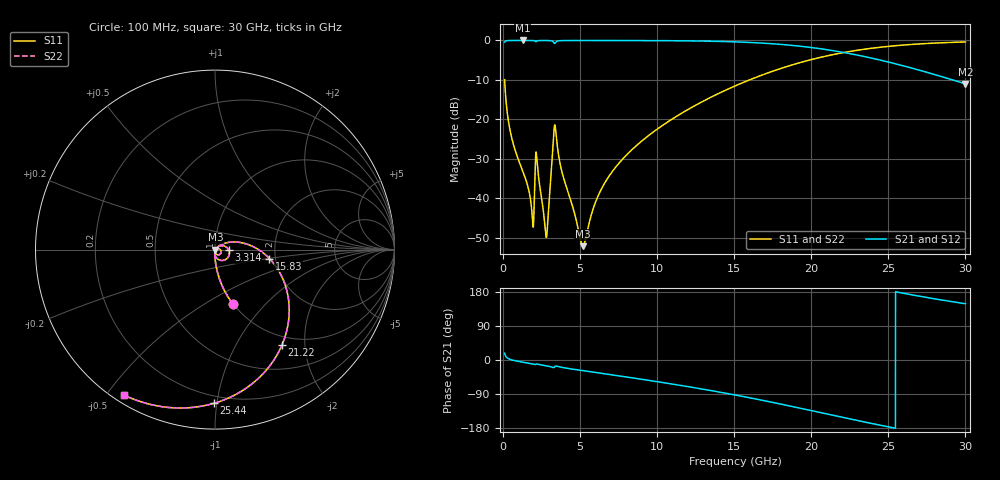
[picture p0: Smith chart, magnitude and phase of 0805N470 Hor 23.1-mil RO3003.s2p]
# GHz S MA R 50
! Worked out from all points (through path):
!   3201 points, 100 MHz to 30 GHz, reference 50 ohm
!   highest |S21| = -0.01 dB at 1.268 GHz (marker M1); lowest = -11.0 dB at 30 GHz (marker M2)
!   group delay of S21, straight-line fit = 20.5 ps
!   lowest |S11| = -52.1 dB at 5.183 GHz (marker M3), VSWR 1.00, Z = 50.2 - j0.114 ohm
!   |S11| at or under -10 dB: 100.6 MHz to 15.99 GHz (15.89 GHz wide, 197 % of centre)
!   |S22| runs from -52.1 to -0.4 dB; largest |S21 - S12| = 0
!   S11 on the Smith chart (normalised r, x): 100 MHz: 0.99, -0.67; 3.314 GHz: 1.17, -0.00; 15.83 GHz: 1.86, -0.20; 21.22 GHz: 0.86, -1.57; 25.44 GHz: 0.15, -0.98; 30 GHz: 0.03, -0.55
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0.1  0.318 -72.0  0.9478 18.0  0.9478 18.0  0.318 -72.0
0.5204688  0.06303 -88.7  0.9974 0.8  0.9974 0.8  0.06303 -88.7
1.267969  0.02233 -93.2  0.9987 -5.7  0.9987 -5.7  0.02233 -93.2
1.884656  0.006208 -76.8  0.9975 -10.0  0.9975 -10.0  0.006208 -76.8
2.230375  0.02534 -76.9  0.9893 -10.9  0.9893 -10.9  0.02534 -76.9
2.800344  0.003204 -27.6  0.9968 -15.2  0.9968 -15.2  0.003204 -27.6
2.921813  0.005849 29.2  0.9958 -16.2  0.9958 -16.2  0.005849 29.2
3.31425  0.07627 -0.7  0.9274 -19.5  0.9274 -19.5  0.07627 -0.7
3.435719  0.06621 -63.8  0.9543 -15.9  0.9543 -15.9  0.06621 -63.8
3.809469  0.02204 -95.1  0.9942 -19.5  0.9942 -19.5  0.02204 -95.1
5.089563  0.002663 -48.1  0.9973 -27.5  0.9973 -27.5  0.002663 -48.1
5.183  0.002479 -27.3  0.9973 -28.1  0.9973 -28.1  0.002479 -27.3
5.995906  0.008915 41.0  0.9973 -32.9  0.9973 -32.9  0.008915 41.0
6.799469  0.01814 44.2  0.997 -37.6  0.997 -37.6  0.01814 44.2
10.06978  0.07688 30.0  0.9934 -57.6  0.9934 -57.6  0.07688 30.0
15.05  0.2649 -3.3  0.9588 -92.3  0.9588 -92.3  0.2649 -3.3
15.83488  0.3075 -9.3  0.9458 -98.4  0.9458 -98.4  0.3075 -9.3
20.03956  0.5743 -44.6  0.811 -133.9  0.811 -133.9  0.5743 -44.6
21.21688  0.6494 -54.9  0.7523 -144.3  0.7523 -144.3  0.6494 -54.9
25.01978  0.8412 -87.1  0.5312 -176.5  0.5312 -176.5  0.8412 -87.1
25.44025  0.8564 -90.4  0.5068 -179.8  0.5068 -179.8  0.8564 -90.4
30  0.9561 -122.0  0.2816 148.5  0.2816 148.5  0.9561 -122.0
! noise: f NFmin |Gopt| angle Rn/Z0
0.1  0.0004286  0.8597  0.7683  0.0006542
3.417  0.03304  0.9357  18.63  0.1116
6.743  0.009976  0.649  36.18  0.004898
10.06  0.01365  0.6314  52.66  0.005656
13.39  0.01791  0.6364  68.06  0.006518
16.7  0.02306  0.6549  82.33  0.007456
20.03  0.02968  0.6841  95.77  0.008547
23.35  0.03866  0.7224  108.6  0.009876
26.67  0.05166  0.7684  121.2  0.01153
30  0.07176  0.8192  133.9  0.01344
